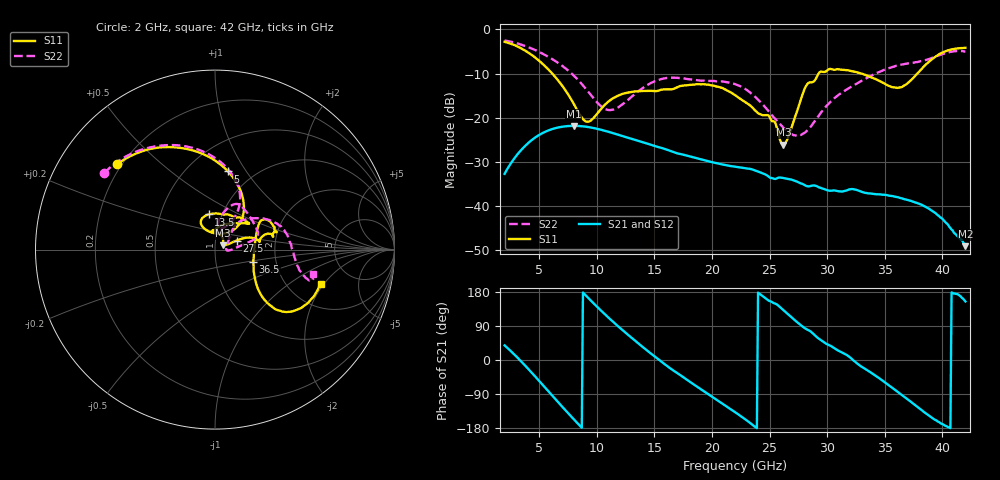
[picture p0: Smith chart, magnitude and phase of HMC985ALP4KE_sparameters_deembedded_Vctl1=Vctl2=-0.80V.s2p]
!s2p File: Measurements: S11, S21, S12, S22
# GHz S dB R 50.0
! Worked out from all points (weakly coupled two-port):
!   401 points, 2 GHz to 42 GHz, reference 50 ohm
!   highest |S21| = -21.86 dB at 8 GHz (marker M1); lowest = -49.1 dB at 42 GHz (marker M2)
!   lowest |S11| = -26.1 dB at 26.2 GHz (marker M3), VSWR 1.10, Z = 54.4 + j2.68 ohm
!   |S11| at or under -10 dB: 6.139 GHz to 29.26 GHz (23.12 GHz wide, 131 % of centre); 32.99 GHz to 37.83 GHz (4.838 GHz wide, 13.7 % of centre)
!   |S22| runs from -24.1 to -2.5 dB; largest |S21 - S12| = 0.00011
!   S11 on the Smith chart (normalised r, x): 2 GHz: 0.18, +0.36; 5 GHz: 0.77, +0.83; 13.5 GHz: 0.86, +0.35; 27.5 GHz: 1.27, +0.13; 36.5 GHz: 1.52, -0.21; 42 GHz: 2.98, -1.87
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2  -2.80 138.8  -32.74 38.5  -32.73 38.5  -2.49 145.3
3.4  -4.23 111.8  -27.45 -2.5  -27.45 -2.5  -3.40 122.7
5  -7.10 80.6  -23.92 -55.2  -23.93 -55.2  -5.09 98.0
6.3  -10.47 57.6  -22.45 -99.6  -22.46 -99.6  -6.99 79.8
8  -16.86 47.8  -21.86 -156.3  -21.86 -156.3  -10.45 62.4
8.7  -20.00 62.8  -21.94 -178.8  -21.95 -178.8  -12.38 59.2
9.4  -20.80 92.0  -22.19 159.4  -22.20 159.4  -14.59 59.4
11  -16.37 118.8  -23.20 112.3  -23.20 112.3  -18.27 75.5
13.5  -14.01 100.4  -25.17 46.4  -25.17 46.4  -14.23 79.3
15.4  -13.84 74.5  -26.71 0.7  -26.71 0.8  -11.40 68.3
18.9  -12.44 38.3  -29.38 -74.3  -29.38 -74.3  -11.54 40.9
22  -14.88 54.4  -31.11 -137.5  -31.12 -137.4  -12.39 16.2
24.9  -19.48 93.3  -33.33 157.2  -33.33 157.2  -18.49 5.3
26.2  -26.12 29.8  -33.70 131.4  -33.69 131.3  -22.29 -3.9
27.5  -17.63 22.6  -34.66 97.3  -34.66 97.1  -24.06 4.0
28.7  -11.96 10.2  -35.42 71.9  -35.44 71.8  -21.58 30.0
31  -9.03 20.9  -36.70 24.4  -36.71 24.3  -14.80 50.1
33.3  -10.29 32.2  -37.07 -23.4  -37.06 -23.3  -11.22 39.4
35.4  -12.83 11.0  -37.70 -67.8  -37.69 -67.7  -8.75 24.5
36.5  -13.04 -17.4  -38.31 -92.8  -38.29 -92.8  -7.93 15.7
39.6  -5.84 -42.6  -42.12 -162.4  -42.15 -162.0  -5.98 -15.5
42  -4.16 -18.2  -49.15 154.6  -49.13 154.5  -4.98 -13.9
